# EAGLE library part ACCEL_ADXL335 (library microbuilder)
ADXL335 Low-Power 3 Axis Accelerometer LFCSP16-R - 16 Pin LFCSP Package (Reflow footprint) LFSCP16-W - 16 Pin LFCSP Package (Wave footprint with extended pads for hand soldering) Digikey: ADXL335BCPZ-RL7CT-ND
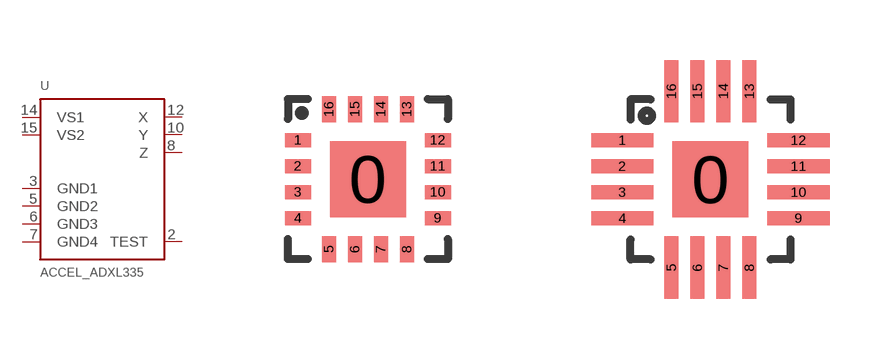
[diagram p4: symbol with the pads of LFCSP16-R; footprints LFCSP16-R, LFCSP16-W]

Designator prefix U

## ACCEL_ADXL335REFLOW  [LFCSP16-R]
2  TEST
3  GND1
5  GND2
6  GND3
7  GND4
8  Z
10  Y
12  X
14  VS1
15  VS2

## ACCEL_ADXL335WAVE  [LFCSP16-W]
Pads as for LFCSP16-R

## Footprint LFCSP16-R (pad centres in mm)
16-Terminal Leadless Frame Chip Scale Package [LFCSP] (CP) - Reflow Footprint Source: Analog Devices .. 780914713ADD8704_0.pdf
smd 1.9 x 1.9: 0 0,0
smd 0.65 x 0.35: 1 -1.75,0.975; 2 -1.75,0.325; 3 -1.75,-0.325; 4 -1.75,-0.975; 9 1.75,-0.975; 10 1.75,-0.325; 11 1.75,0.325; 12 1.75,0.975
smd 0.35 x 0.65: 5 -0.975,-1.75; 6 -0.325,-1.75; 7 0.325,-1.75; 8 0.975,-1.75; 13 0.975,1.75; 14 0.325,1.75; 15 -0.325,1.75; 16 -0.975,1.75

## Footprint LFCSP16-W (pad centres in mm)
16-Terminal Leadless Frame Chip Scale Package [LFCSP] (CP) - Wave Footprint Source: Analog Devices .. 780914713ADD8704_0.pdf
smd 1.9 x 1.9: 0 0,0
smd 1.558 x 0.35: 1 -2.204,0.975; 2 -2.204,0.325; 3 -2.204,-0.325; 4 -2.204,-0.975; 9 2.204,-0.975; 10 2.204,-0.325; 11 2.204,0.325; 12 2.204,0.975
smd 0.35 x 1.558: 5 -0.975,-2.204; 6 -0.325,-2.204; 7 0.325,-2.204; 8 0.975,-2.204; 13 0.975,2.204; 14 0.325,2.204; 15 -0.325,2.204; 16 -0.975,2.204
